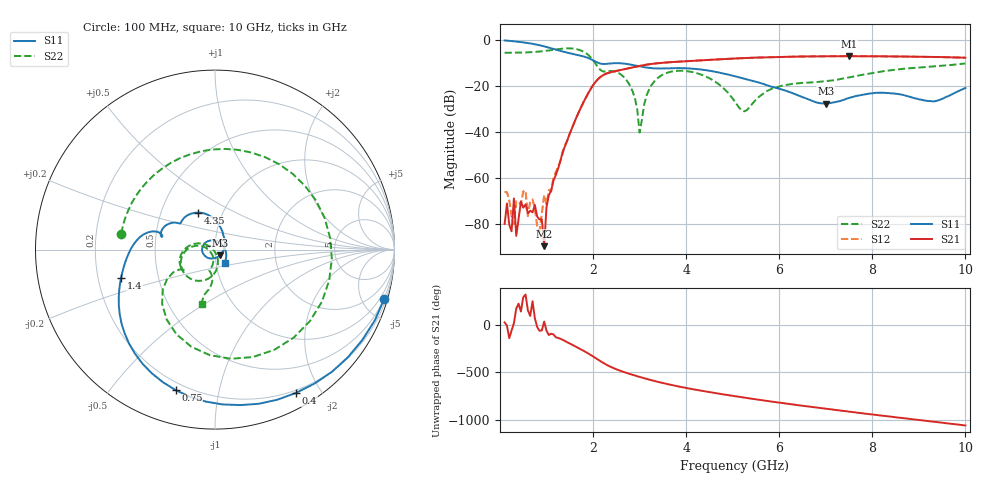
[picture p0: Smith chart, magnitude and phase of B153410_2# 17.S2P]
!  2-Port S-parameters saved by WinCal
! VAR MeasName=S-Parameters (CALIBRATED_DATA) read from VNA (N5245A)
! VAR MeasDate=2016-12-23 10:00:13
! VAR NAME=B153410_2# 17
! VAR FILENAME=B153410_2# 17.S2P
! VAR DATE=2016-12-23 10:00:13
! VAR PHYS_PORTS=1,2
# Hz S DB R 50
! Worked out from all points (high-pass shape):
!   199 points, 100 MHz to 10 GHz, reference 50 ohm
!   highest |S21| = -6.96 dB at 7.5 GHz (marker M1); lowest = -89.5 dB at 950 MHz (marker M2)
!   |S21| within 3 dB of the highest: 3.429 GHz to end of sweep
!   lowest |S11| = -27.5 dB at 7 GHz (marker M3), VSWR 1.09, Z = 52.8 - j3.31 ohm
!   |S11| at or under -10 dB: 2.126 GHz to end of sweep
!   |S22| runs from -40.2 to -3.6 dB; largest |S21 - S12| = 0.0031
!   S11 on the Smith chart (normalised r, x): 100 MHz: 0.46, -7.01; 400 MHz: 0.17, -1.70; 750 MHz: 0.16, -0.75; 1.4 GHz: 0.30, -0.14; 4.35 GHz: 0.76, +0.33; 10 GHz: 1.10, -0.16
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1e8  -0.16 -16.2  -79.89 24.7  -65.99 -88.2  -5.52 170.3
1.5e8  -0.23 -23.9  -70.95 -8.5  -66.01 87.7  -5.51 165.3
2.5e8  -0.42 -39.0  -83.02 -59.5  -76.37 -65.9  -5.51 155.4
3e8  -0.52 -46.3  -68.74 16.1  -79.98 -172.8  -5.48 150.3
4e8  -0.75 -60.5  -77.78 -138.2  -70.02 -63.2  -5.45 139.8
4.5e8  -0.86 -67.4  -70.06 138.9  -71.44 2.7  -5.43 134.3
7.5e8  -1.80 -105.7  -71.57 68.2  -73.04 129.4  -5.15 98.3
8.5e8  -2.22 -117.0  -77.89 -63.0  -82.93 171.2  -4.98 84.4
9.5e8  -2.72 -127.6  -89.48 33.3  -67.28 -51.9  -4.76 69.3
1.4e9  -5.23 -163.0  -45.98 -170.8  -45.44 -171.8  -3.62 -15.2
1.75e9  -6.83 176.6  -28.85 99.2  -28.86 99.4  -4.60 -92.8
2.75e9  -10.43 152.5  -12.29 -150.4  -12.28 -150.5  -18.27 164.9
3e9  -11.41 146.0  -11.20 172.4  -11.22 172.2  -40.18 -178.0
3.15e9  -11.94 144.4  -10.67 151.7  -10.68 151.6  -24.07 -74.8
3.4e9  -12.32 142.7  -10.03 120.0  -10.02 119.8  -16.31 -98.1
4.35e9  -12.86 115.0  -8.75 25.7  -8.77 25.6  -15.21 -174.0
5.05e9  -15.72 89.4  -7.98 -30.1  -8.00 -30.1  -26.79 172.5
6.7e9  -26.33 -1.8  -7.05 -143.0  -7.07 -142.9  -18.36 -105.0
7e9  -27.54 -48.2  -7.00 -161.8  -7.01 -161.7  -17.82 -101.5
7.5e9  -25.13 -116.7  -6.96 167.7  -6.98 167.7  -16.21 -96.0
8.35e9  -22.98 167.6  -7.10 117.8  -7.09 117.9  -13.20 -98.1
1e10  -20.79 -54.4  -7.65 23.1  -7.67 23.3  -10.13 -103.7
